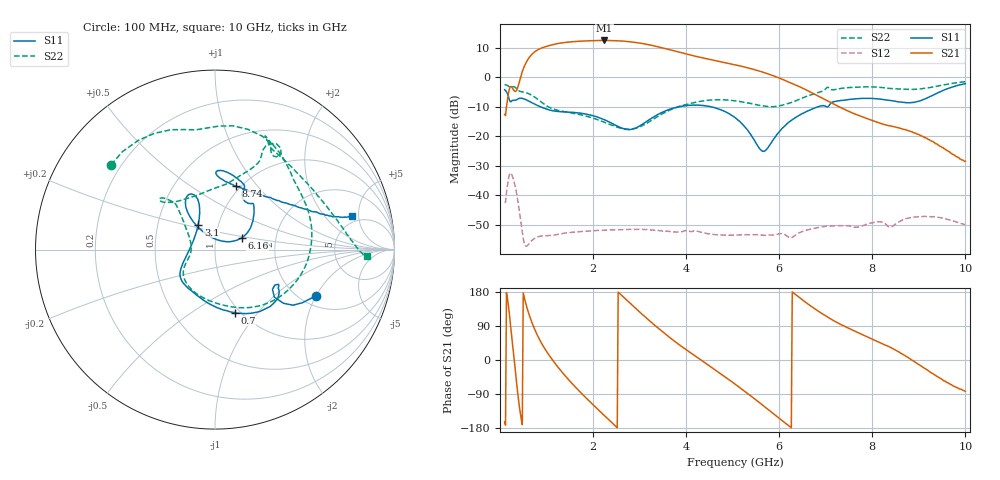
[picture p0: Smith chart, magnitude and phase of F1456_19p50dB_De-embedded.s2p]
! Integrated Device Technology
! Corporate Headquarters
! 6024 Silver Creek Valley Road
! San Jose, CA 95138  USA
! Phone:  1-408-284-8200
! Toll Free:  1-800-223-1366
! Webpage:  http://www.idt.com/
! Timing and RF Division
! 515 Groton Road, Suite 102
! Westford, MA 01886-6024
! Device:  F1456
! Description: 6-bit 0.5 dB Transmit Variable Gain Amplifier
! Frequency:  2100.0 -  2950.00 MHz
! Package:  6x6 mm Thin QFN Plastic Package: 28 pin
! State:  39
! Atten State:  19.5 dB
! Voltage:  +5.00 Volts
! Current:  216.965 mA
! Data:  The device was measured on a the F1455 evaluation board which has
!  individual transmission lines to the RF pins.  Data was collected
!  using a calibrated network analyzer.  The evaluation board was
!  de-embedded using a TRL calibration technique.
!  The reference plane is the edge of the package pin.
!  Pin  1 = CSb
!  Pin  2 = DATA
!  Pin  3 = CLK
!  Pin  4 = RSET
!  Pin  5 = GND
!  Pin  6 = RFIN  = Port 1
!  Pin  7 = GND
!  Pin  8 = NC
!  Pin  9 = NC
!  Pin 10 = NC
!  Pin 11 = NC
!  Pin 12 = NC
!  Pin 13 = NC
!  Pin 14 = /STBY
!  Pin 15 = GND
!  Pin 16 = RFOUT  = Port 2
!  Pin 17 = GND
!  Pin 18 = NC
!  Pin 19 = NC
!  Pin 20 = NC
!  Pin 21 = GND
!  Pin 22 = NC
!  Pin 23 = GND
!  Pin 24 = NC
!  Pin 25 = NC
!  Pin 26 = NC
!  Pin 27 = GND
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# GHz S dB R 50
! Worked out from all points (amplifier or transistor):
!   496 points, 100 MHz to 10 GHz, reference 50 ohm
!   highest |S21| = 12.5 dB at 2.24 GHz (marker M1)
!   |S21| within 3 dB of that: 832.2 MHz to 3.616 GHz (2.783 GHz wide, 125 % of centre)
!   unconditionally stable (mu >= 1): start of sweep to end of sweep
!   at 1.74 GHz: K = 44.19, MAG = 12.8 dB, |S12| = -52.2 dB
!   at 5.06 GHz: K = 116.50, MAG = 5.2 dB, |S12| = -53.5 dB
!   at 10 GHz: K = 452.46, MAG = -18.8 dB, |S12| = -49.9 dB
!   S11 on the Smith chart (normalised r, x): 100 MHz: 2.36, -2.00; 700 MHz: 0.94, -0.76; 3.1 GHz: 0.80, +0.23; 6.16 GHz: 1.33, +0.18; 8.74 GHz: 0.95, +0.78; 10 GHz: 4.19, +4.08
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0.1  -4.18 -25.0  -12.55 -163.2  -42.29 48.9  -2.54 140.8
0.22  -8.21 -34.5  -3.19 100.2  -32.39 -50.8  -3.41 99.1
0.3  -7.72 -30.8  -4.39 8.6  -35.21 -134.4  -3.17 74.6
0.42  -7.08 -37.6  -1.24 -125.8  -45.72 141.7  -4.65 41.4
0.56  -7.57 -56.6  4.97 146.9  -57.20 148.3  -5.17 11.7
0.7  -8.71 -72.7  8.05 94.7  -55.06 142.7  -6.20 -19.8
0.94  -10.41 -97.0  10.21 34.5  -53.72 98.9  -8.97 -65.5
1.18  -11.42 -115.6  11.26 -8.3  -53.41 72.8  -10.87 -96.3
1.48  -11.77 -131.7  11.98 -52.7  -52.61 49.6  -11.88 -123.2
1.76  -12.19 -142.2  12.30 -89.1  -52.21 32.6  -12.74 -139.1
2.24  -14.33 -157.7  12.52 -146.2  -51.80 8.7  -15.18 -156.4
2.64  -17.32 173.6  12.30 167.5  -51.58 -9.7  -17.37 -174.1
3.1  -15.49 123.8  11.36 115.7  -51.52 -31.8  -16.01 154.2
3.4  -12.51 111.3  10.37 83.9  -51.85 -46.0  -13.19 140.3
3.74  -10.37 109.3  9.00 50.6  -52.36 -59.5  -10.45 132.5
4.1  -9.42 113.6  7.53 18.7  -52.22 -76.4  -8.80 131.9
5.06  -13.73 127.9  4.25 -64.4  -53.49 -123.5  -7.94 138.1
6.16  -15.80 24.0  -1.29 -169.4  -53.72 165.4  -9.00 85.0
6.7  -10.77 41.7  -5.21 140.5  -51.32 144.2  -5.82 64.8
8.36  -7.74 88.0  -16.36 35.3  -50.67 70.2  -3.72 62.4
8.74  -8.59 72.0  -17.90 8.2  -47.82 66.6  -4.05 49.1
10  -2.11 13.8  -28.41 -82.4  -49.92 -22.6  -1.46 -2.6
